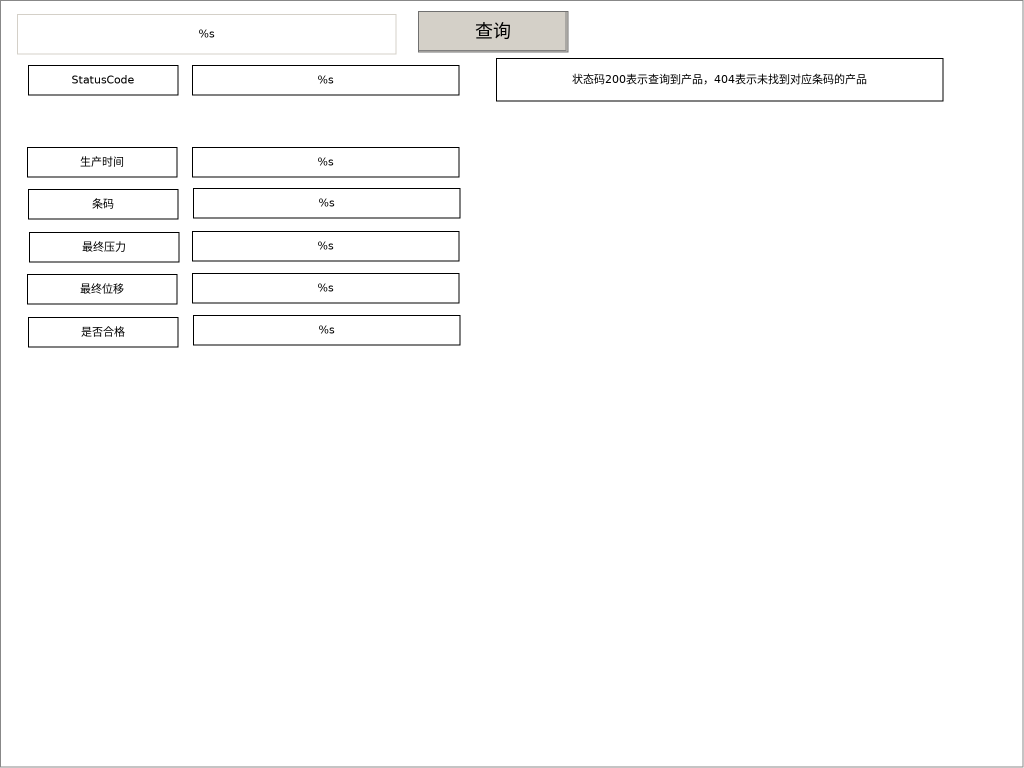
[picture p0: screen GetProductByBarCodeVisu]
VISUALIZATION GetProductByBarCodeVisu  // 1024x768
    Button (418,11 150x41), "查询"
        tap MAIN.fbGetProductByBarCode.bSend
    Textfield (17,14 379x40), "%s", text variable: MAIN.fbGetProductByBarCode.sBarCode
        OnMouseClick: write the text variable via Default
    Rectangle (28,65 150x30), "StatusCode"
    Rectangle (27,147 150x30), "生产时间"
    Rectangle (28,189 150x30), "条码"
    Rectangle (29,232 150x30), "最终压力"
    Rectangle (27,274 150x30), "最终位移"
    Rectangle (28,317 150x30), "是否合格"
    Rectangle (192,147 267x30), "%s", text variable: MAIN.fbGetProductByBarCode.product.CreatDateTime
    Rectangle (193,188 267x30), "%s", text variable: MAIN.fbGetProductByBarCode.product.BarCode
    Rectangle (192,231 267x30), "%s", text variable: MAIN.fbGetProductByBarCode.product.FinalPressure
    Rectangle (192,273 267x30), "%s", text variable: MAIN.fbGetProductByBarCode.product.FinalDisplacement
    Rectangle (193,315 267x30), "%s", text variable: MAIN.fbGetProductByBarCode.product.IsQualified
    Rectangle (192,65 267x30), "%s", text variable: MAIN.fbGetProductByBarCode.nStatusCode
    Rectangle (496,58 447x43), "状态码200表示查询到产品，404表示未找到对应条码的产品"
END_VISUALIZATION
